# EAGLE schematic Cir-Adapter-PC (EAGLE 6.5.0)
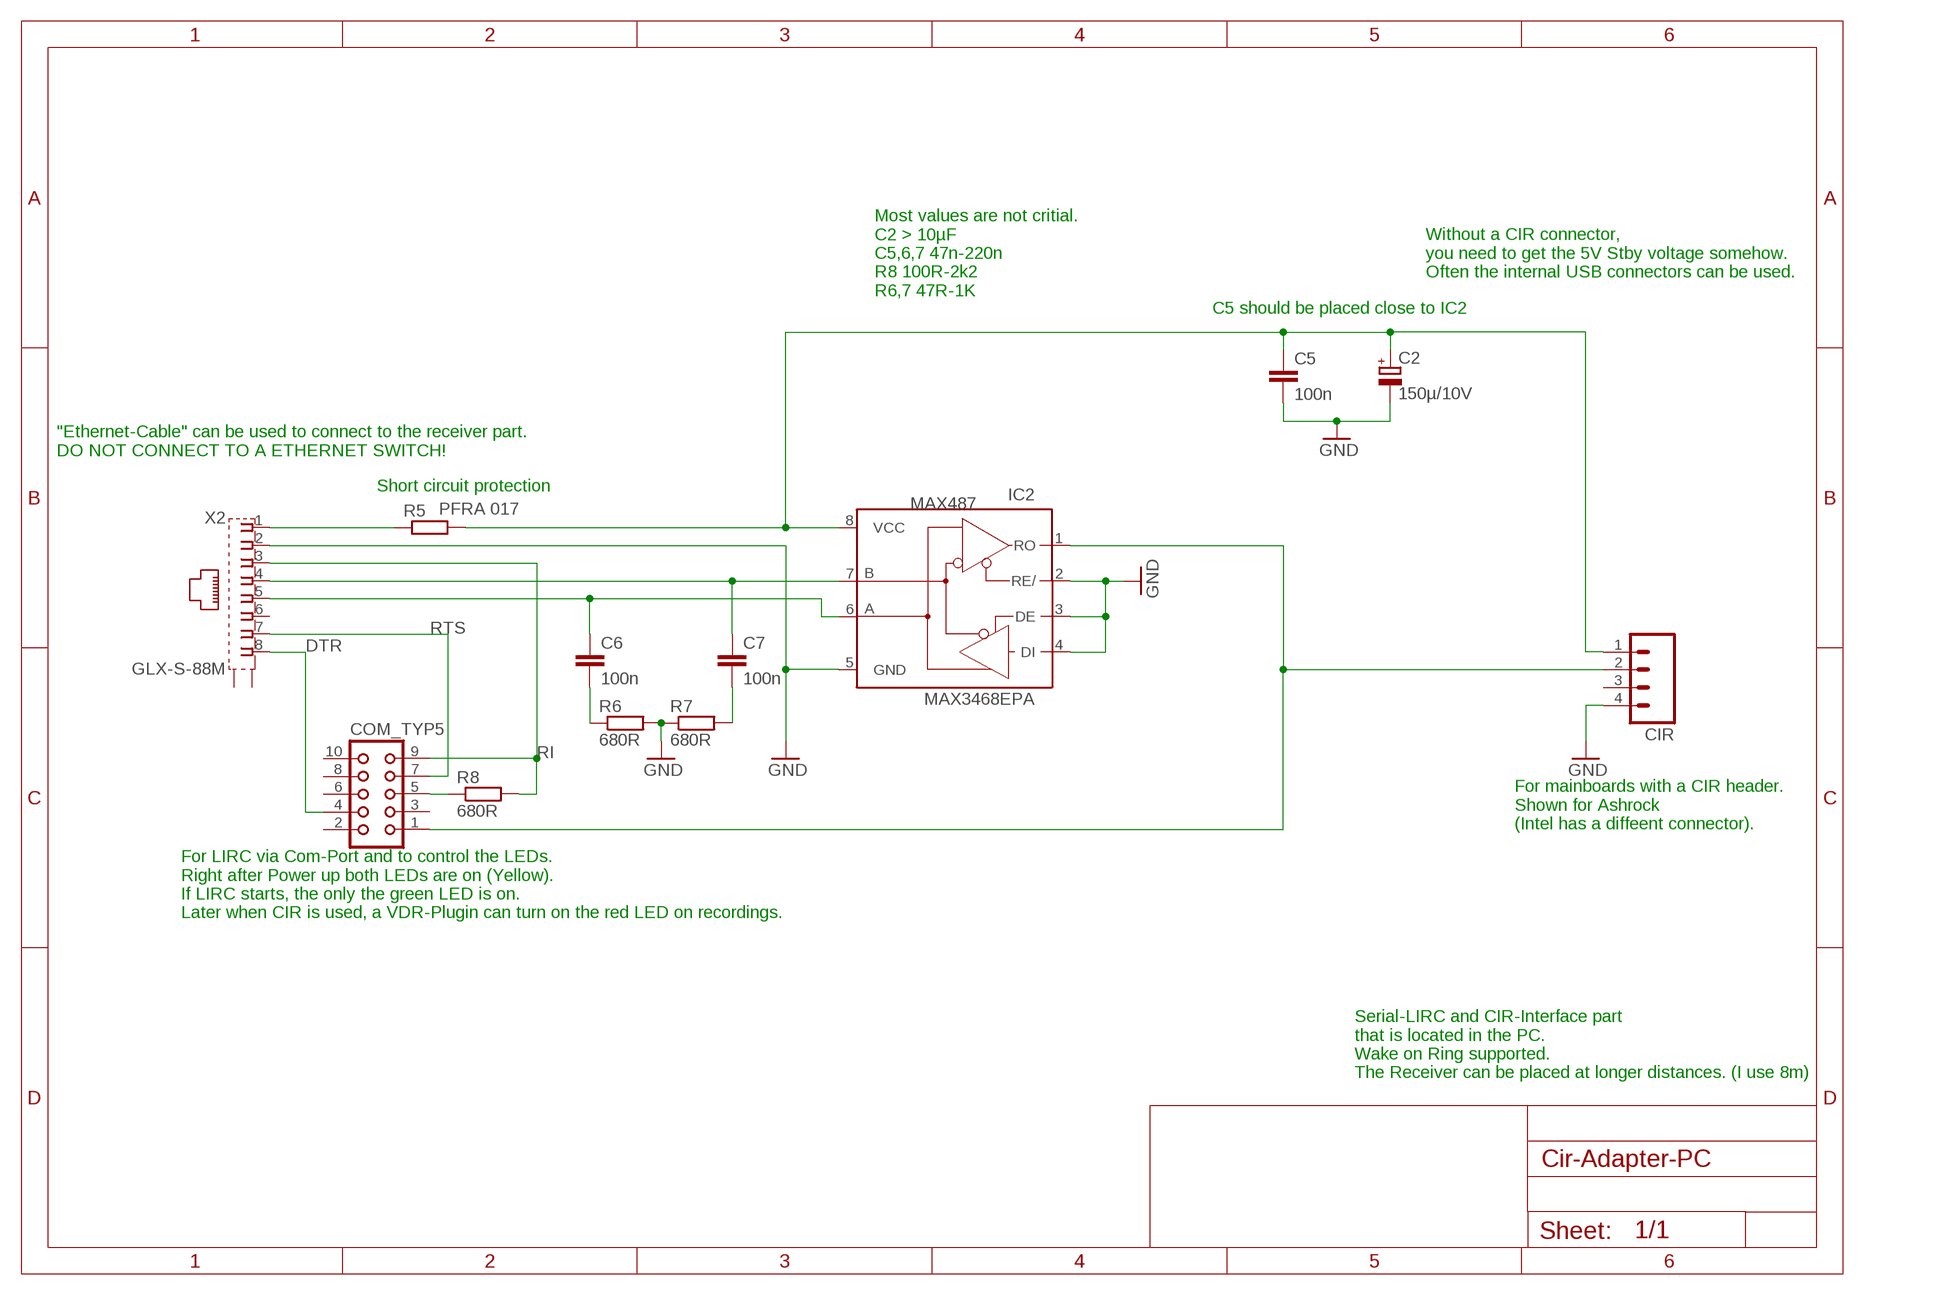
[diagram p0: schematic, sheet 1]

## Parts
C2  150µ/10V  CPOL-EUE2.5-5  [E2,5-5]
C5  100n  C2,5-3  [C2.5-3]
C6  100n  C2,5-3  [C2.5-3]
C7  100n  C2,5-3  [C2.5-3]
CIR  MA04  [04PA]
COM_TYP5  CON10  [CON10]
IC2  MAX3468EPA  [DIL08]
R5  PFRA 017  R-EU_0207/10  [0207/10]
R6  680R  R-EU_0207/10  [0207/10]
R7  680R  R-EU_0207/10  [0207/10]
R8  680R  R-EU_0207/10  [0207/10]
X2  GLX-S-88M  [GLX-S-88M]

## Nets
DTR: COM_TYP5.4 X2.8
GND: C2.- C5.2 CIR.4 IC2.2(RE/) IC2.3(DE) IC2.4(DI) IC2.5(GND) R6.2 R7.1 X2.2
N$13: C7.1 IC2.7(B) X2.4
N$14: C6.1 IC2.6(A) X2.5
N$15: R5.1 X2.1
N$16: C2.+ C5.1 CIR.1 IC2.8(VCC) R5.2
N$18: COM_TYP5.5 R8.1
N$19: C7.2 R7.2
N$20: C6.2 R6.1
N$25: CIR.2 COM_TYP5.1 IC2.1(RO)
RI: COM_TYP5.9 R8.2 X2.3
RTS: COM_TYP5.7 X2.7
Unconnected: CIR.3 COM_TYP5.2 COM_TYP5.3 COM_TYP5.6 COM_TYP5.8 COM_TYP5.10 X2.6 X2.S1 X2.S2

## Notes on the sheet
- Most values are not critial.
  C2 > 10µF
  C5,6,7 47n-220n
  R8 100R-2k2
  R6,7 47R-1K
- Without a CIR connector,
  you need to get the 5V Stby voltage somehow.
  Often the internal USB connectors can be used.
- C5 should be placed close to IC2
- "Ethernet-Cable" can be used to connect to the receiver part.
  DO NOT CONNECT TO A ETHERNET SWITCH!
- Short circuit protection
- For mainboards with a CIR header.
  Shown for Ashrock
  (Intel has a diffeent connector).
- For LIRC via Com-Port and to control the LEDs.
  Right after Power up both LEDs are on (Yellow).
  If LIRC starts, the only the green LED is on.
  Later when CIR is used, a VDR-Plugin can turn on the red LED on recordings.
- Serial-LIRC and CIR-Interface part
  that is located in the PC.
  Wake on Ring supported.
  The Receiver can be placed at longer distances. (I use 8m)

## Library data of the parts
C2 = rcl:CPOL-EU: POLARIZED CAPACITOR, European symbol
C5-C7 = capacitor-wima:C: CAPACITOR
CIR = con-amp-quick:MA04: AMP QUICK CONNECTOR; OC_FARNELL: unknown; OC_NEWARK: unknown
COM_TYP5 = con-harting:CON10: CONNECTOR; OC_FARNELL: unknown; OC_NEWARK: unknown
IC2 = maxim:MAX34*: +5V, Fail-Safe, 40Mbps, Profibus RS-485/RS-422 Transceivers Source: MAX3465-MAX3469.pdf; MPN: MAX487; OC_FARNELL: unknown
R5-R8 = resistor:R-EU_: RESISTOR, European symbol
X2 = con-kycon:GLX-S-88M: Mod. Jack, Right Angle, 8 posiotion, 8 contatcs RJ45 Source: GLX-S-88M.pdf; OC_FARNELL: unknown; OC_NEWARK: unknown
